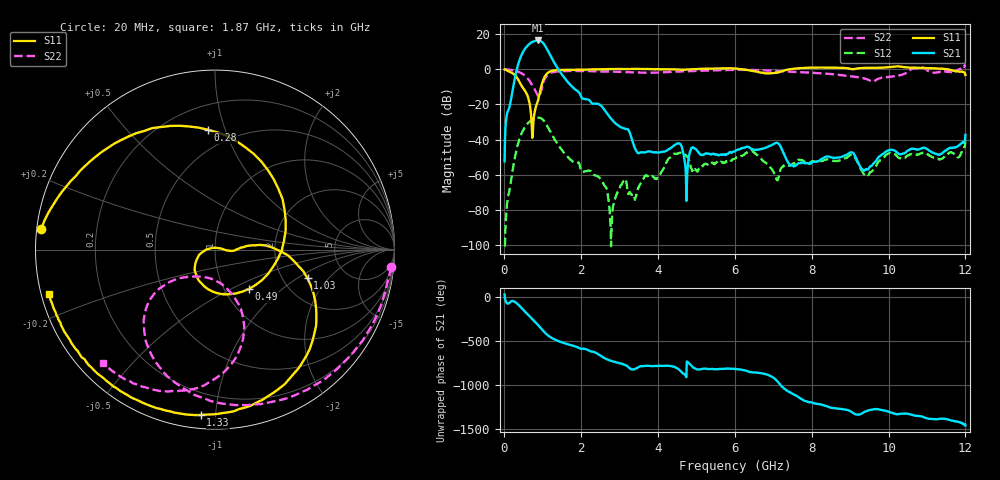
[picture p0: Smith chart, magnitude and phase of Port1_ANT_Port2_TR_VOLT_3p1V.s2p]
! Created Mon Aug 25 11:19:48 2025
# hz S ma R 50
! 2 Port Network Data from SP1.SP block
! freq  magS11  angS11  magS21  angS21  magS12  angS12  magS22  angS22
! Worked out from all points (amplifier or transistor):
!   1200 points, 10 MHz to 12 GHz, reference 50 ohm
!   highest |S21| = 16.3 dB at 870 MHz (marker M1)
!   |S21| within 3 dB of that: 604.4 MHz to 1.062 GHz (457.7 MHz wide, 54.9 % of centre)
!   unconditionally stable (mu >= 1): start of sweep to 2.671 GHz; 3.879 GHz to 4.98 GHz; 6.17 GHz to 7.451 GHz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
!   at 2.01 GHz: K = 42.98, MAG = 1.7 dB, |S12| = -58.1 dB
!   at 6.01 GHz: K = -236.92, MSG = 2.1 dB, |S12| = -50.7 dB
!   at 12 GHz: K = -1632.68, MSG = 1.5 dB, |S12| = -40.3 dB
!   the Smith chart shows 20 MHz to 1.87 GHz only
!   S11 on the Smith chart (normalised r, x): 20 MHz: 0.01, +0.06; 280 MHz: 0.36, +0.87; 490 MHz: 1.30, -0.62; 1.03 GHz: 2.72, -1.23; 1.33 GHz: 0.07, -0.91; 1.87 GHz: 0.02, -0.13
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1e7  0.9818 176.4  0.002446 28.9  1.009e-05 146.4  0.99 -3.2
2e7  0.9744 173.1  0.01007 -13.7  9.854e-06 -132.4  0.985 -5.8
2.8e8  0.669 93.4  0.5843 -56.1  0.003234 157.0  0.9023 -71.1
3.8e8  0.4694 36.6  1.571 -92.5  0.009135 118.3  0.8322 -94.0
4.9e8  0.2897 -49.2  3.079 -142.8  0.01842 67.6  0.7163 -116.5
5.8e8  0.2034 -111.6  4.292 176.3  0.02621 27.2  0.5892 -132.1
6.6e8  0.1061 -155.4  5.234 140.6  0.03245 -7.9  0.46 -142.3
7.7e8  0.04352 4.4  6.158 91.3  0.03894 -56.0  0.297 -143.9
8.7e8  0.1199 0.3  6.499 45.6  0.04194 -100.4  0.1795 -123.3
9.5e8  0.2804 4.8  6.221 6.6  0.04086 -138.3  0.2228 -73.5
1.03e9  0.5397 -17.2  5.185 -33.1  0.03458 -176.9  0.4573 -69.1
1.17e9  0.8311 -60.1  2.815 -88.2  0.01931 130.3  0.7446 -93.1
1.33e9  0.9248 -95.0  1.355 -127.7  0.009458 94.3  0.8466 -111.5
1.87e9  0.9571 -164.8  0.2542 153.7  0.00217 46.3  0.885 -134.6
2.01e9  0.9602 -174.1  0.1589 129.6  0.001249 27.9  0.8846 -136.9
2.79e9  1.003 174.1  0.03819 -9.3  2.715e-05 121.3  0.8539 -148.7
4.01e9  0.9946 177.1  0.004308 -66.1  0.0008292 54.6  0.8007 141.9
6.01e9  1.034 145.8  0.004733 -100.3  0.002924 -41.5  0.9522 125.0
8.01e9  1.101 71.0  0.002292 -124.4  0.00245 -96.0  0.787 141.6
1.001e10  1.136 -176.4  0.005013 130.9  0.004083 129.9  0.6018 103.6
1.099e10  1.067 -137.2  0.005575 57.5  0.004071 46.8  0.96 66.5
1.2e10  0.6769 -71.5  0.01358 -25.1  0.009669 -51.4  1.339 -171.9
